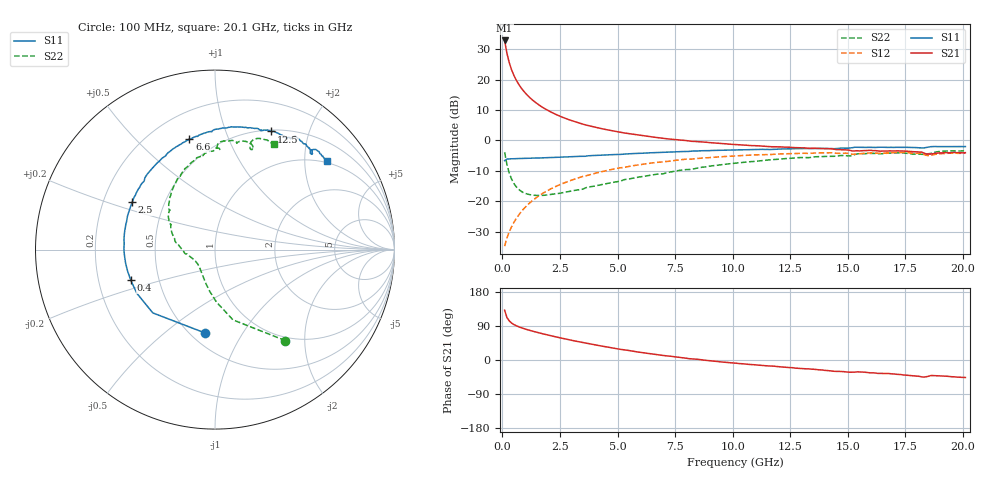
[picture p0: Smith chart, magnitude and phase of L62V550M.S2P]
!  Infineon Technologies AG
! BFR380L3 , PF131585-7, No.6, Th 09.10.01, soldered on pcb-board, measured with PP GSG850
!  Vce=2.5 V,  Ic=50.0 mA
! Common Emitter S-Parameters:  15. November 2001
#  GHz  S  MA  R  50
! f  S11  S21  S12  S22
! GHz  Mag  Ang  Mag  Ang  Mag  Ang  Mag  Ang
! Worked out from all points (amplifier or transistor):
!   201 points, 100 MHz to 20.1 GHz, reference 50 ohm
!   highest |S21| = 32.9 dB at 100 MHz (marker M1)
!   |S21| within 3 dB of that: start of sweep to 171.4 MHz
!   unconditionally stable (mu >= 1): 910.6 MHz to 4.306 GHz
!   at 3.4 GHz: K = 1.02, MAG = 8.0 dB, |S12| = -12.0 dB
!   at 10.1 GHz: K = 0.96, MSG = 1.9 dB, |S12| = -5.1 dB
!   at 20.1 GHz: K = 0.99, MSG = 0.1 dB, |S12| = -4.2 dB
!   S11 on the Smith chart (normalised r, x): 100 MHz: 0.59, -0.70; 400 MHz: 0.34, -0.16; 2.5 GHz: 0.32, +0.24; 6.6 GHz: 0.36, +0.73; 12.5 GHz: 0.52, +1.46; 20.1 GHz: 0.96, +2.56
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0.1  0.4677 -96.8  43.91 131.6  0.01838 59.7  0.6411 -52.3
0.2  0.4944 -134.5  27.08 112.1  0.02503 58.4  0.4042 -75.6
0.3  0.4989 -150.7  19.05 103.2  0.03154 60.8  0.2925 -88.4
0.4  0.4994 -159.9  14.59 97.7  0.03806 63.3  0.2332 -97.4
0.5  0.5016 -166.4  11.79 93.7  0.04497 65.5  0.1974 -104.6
0.6  0.5038 -171.2  9.881 90.6  0.05182 67.0  0.1745 -110.6
0.7  0.5048 -175.2  8.511 88.0  0.05877 68.1  0.1591 -115.7
0.8  0.5065 -178.2  7.472 85.6  0.06617 68.9  0.1481 -120.4
1  0.5068 176.4  6.01 81.6  0.08064 69.6  0.135 -128.0
1.3  0.5126 170.0  4.655 76.3  0.1025 69.3  0.1268 -137.0
1.6  0.5163 164.2  3.809 71.5  0.1245 68.4  0.1252 -144.0
2  0.5235 157.7  3.085 65.6  0.1529 66.4  0.1282 -151.5
2.5  0.5323 150.0  2.506 58.6  0.1883 63.4  0.1361 -159.2
3.5  0.5489 136.3  1.853 45.9  0.2566 56.6  0.159 -171.2
5  0.5895 118.8  1.391 29.5  0.3497 45.7  0.2112 170.8
6.6  0.6323 103.0  1.131 14.8  0.4321 34.3  0.2762 153.2
6.8  0.6358 101.1  1.106 13.3  0.4417 32.8  0.2815 151.0
10.1  0.6996 77.1  0.8587 -8.2  0.5572 11.0  0.4239 122.4
12.5  0.7297 64.5  0.7716 -20.2  0.61 -3.6  0.5098 103.2
13.5  0.7371 60.0  0.7455 -24.4  0.6196 -9.4  0.5336 96.7
16.8  0.7716 47.8  0.6743 -35.8  0.6253 -25.2  0.6209 76.5
20.1  0.7944 38.4  0.6304 -46.2  0.6196 -38.7  0.6765 60.8
